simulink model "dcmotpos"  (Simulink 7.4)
settings: Solver=ode15s  StartTime=0.0  StopTime=0.1  MaxStep=1e-3  RelTol=1e-3

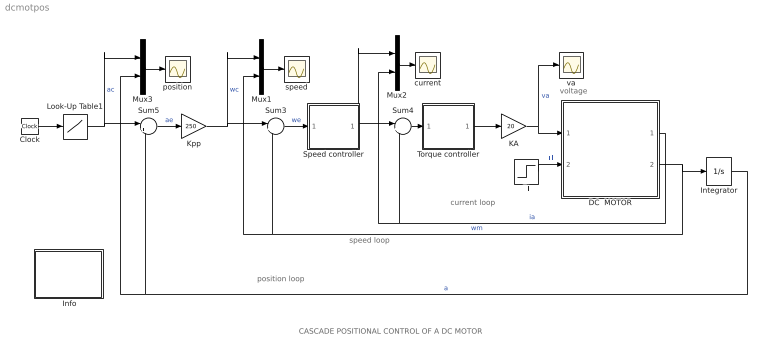
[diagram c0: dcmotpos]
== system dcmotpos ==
  note: voltage
  note: speed loop
  note: current loop
  note: position loop
  note: CASCADE POSITIONAL CONTROL OF A DC MOTOR
  " Info" : Subsystem
  Clock : Clock
  DC  MOTOR : Subsystem  mask{Ra=2.0, La=5.2e-3, J=1.5e-4, Bm=1e-3, K=0.1}
      mask prompts: Ra "Armature resistance [ohm]"; La "Armature inductance [H]"; J "Moment of inertia [Kg.m^2]"; Bm "Frictional torque cefficient"; K "Electromechanical coupling coefficient [N.m/A]"
      mask help: Block diagram of a dc motor with constant fiield excitation.
  Integrator : Integrator
  KA : Gain  Gain=20  ParameterDataType=sfix(16)  ParameterScaling=2^0  OutDataType=sfix(16)  OutScaling=2^0
  Kpp : Gain  Gain=250  ParameterDataType=sfix(16)  ParameterScaling=2^0  OutDataType=sfix(16)  OutScaling=2^0
  Look-Up Table1 : Lookup  InputValues="[0  .05  .05 1]"  Table="[1 1 .5  .5]"  OutDataType=sfix(16)  OutScaling=2^0
  Mux1 : Mux  Inputs=2
  Mux2 : Mux  Inputs=2
  Mux3 : Mux  Inputs=2
  Speed controller : Subsystem  mask{Kp=1.17, Ki=527, sat=18}
      mask prompts: Kp "Proportional gain (Kp)"; Ki "Integral gain (Ki)"; sat "Saturation limit [pu]"
      mask help: Proportional-Integral Speed Controller
  Sum3 : Sum  Inputs=|+-  OutDataType=sfix(16)  OutScaling=2^0
  Sum4 : Sum  Inputs=|+-  OutDataType=sfix(16)  OutScaling=2^0
  Sum5 : Sum  Inputs=|+-  OutDataType=sfix(16)  OutScaling=2^0
  Tl : Step  Time=0.04  After=0.38  SampleTime=0
  Torque controller : Subsystem  mask{Kp=1.38, Ki=5880, sat=3}
      mask prompts: Kp "Proportional gain (Kp)"; Ki "Integral gain (Ki)"; sat "Saturation limit [pu]"
      mask help: Proportional-Integral Speed Controller
  current : Scope
  position : Scope
  speed : Scope
  va : Scope
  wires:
  Tl/1 -> DC  MOTOR/2(Tl)  "Tl"
  Mux1/1 -> speed/1
  Mux2/1 -> current/1
  Kpp/1 -> Sum3/1, Mux1/1  "wc"
  DC  MOTOR/1(ia) -> Sum4/2, Mux2/2  "ia"
  Sum5/1 -> Kpp/1  "ae"
  Clock/1 -> Look-Up Table1/1
  Mux3/1 -> position/1
  Look-Up Table1/1 -> Sum5/1, Mux3/1  "ac"
  Integrator/1 -> Sum5/2, Mux3/2  "a"
  Speed controller/1(c) -> Sum4/1, Mux2/1
  Sum3/1 -> Speed controller/1(er)  "we"
  Sum4/1 -> Torque controller/1(er)
  Torque controller/1(c) -> KA/1
  KA/1 -> va/1, DC  MOTOR/1(va)  "va"
  DC  MOTOR/2(wm) -> Integrator/1, Sum3/2, Mux1/2  "wm"

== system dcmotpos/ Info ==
  note: This demo simulates the cascade control of a DC motor drive for position control

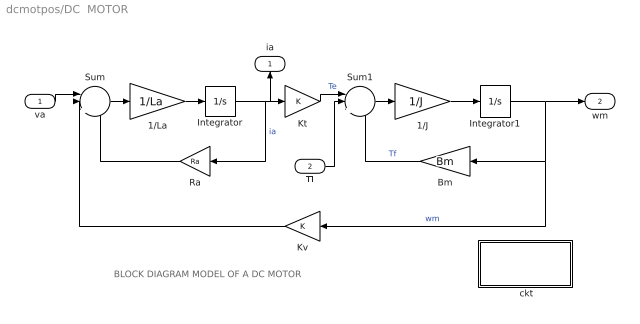
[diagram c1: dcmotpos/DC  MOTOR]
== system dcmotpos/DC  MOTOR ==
  note: BLOCK DIAGRAM MODEL OF A DC MOTOR
  va : Inport  OutDataType=sfix(16)  OutScaling=2^0
  Tl : Inport  Port=2  OutDataType=sfix(16)  OutScaling=2^0
  " ckt" : Subsystem
  1/J : Gain  Gain=1/J  ParameterDataType=sfix(16)  ParameterScaling=2^0  OutDataType=sfix(16)  OutScaling=2^0
  1/La : Gain  Gain=1/La  ParameterDataType=sfix(16)  ParameterScaling=2^0  OutDataType=sfix(16)  OutScaling=2^0
  Bm : Gain  Gain=Bm  ParameterDataType=sfix(16)  ParameterScaling=2^0  OutDataType=sfix(16)  OutScaling=2^0
  Integrator : Integrator
  Integrator1 : Integrator
  Kt : Gain  Gain=K  ParameterDataType=sfix(16)  ParameterScaling=2^0  OutDataType=sfix(16)  OutScaling=2^0
  Kv : Gain  Gain=K  ParameterDataType=sfix(16)  ParameterScaling=2^0  OutDataType=sfix(16)  OutScaling=2^0
  Ra : Gain  Gain=Ra  ParameterDataType=sfix(16)  ParameterScaling=2^0  OutDataType=sfix(16)  OutScaling=2^0
  Sum : Sum  Inputs=||+--  OutDataType=sfix(16)  OutScaling=2^0
  Sum1 : Sum  Inputs=||+--  OutDataType=sfix(16)  OutScaling=2^0
  ia : Outport
  wm : Outport  Port=2
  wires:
  Kv/1 -> Sum/2
  Ra/1 -> Sum/3
  Kt/1 -> Sum1/1  "Te"
  Bm/1 -> Sum1/3  "Tf"
  Sum/1 -> 1/La/1
  1/La/1 -> Integrator/1
  Integrator/1 -> Ra/1, Kt/1, ia/1  "ia"
  Sum1/1 -> 1/J/1
  1/J/1 -> Integrator1/1
  va/1 -> Sum/1
  Tl/1 -> Sum1/2
  Integrator1/1 -> Bm/1, Kv/1, wm/1  "wm"

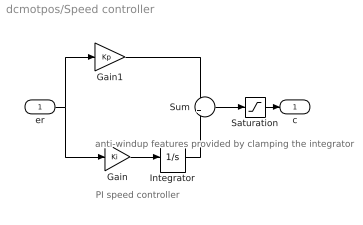
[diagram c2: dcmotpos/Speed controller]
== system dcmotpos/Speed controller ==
  note: anti-windup features provided by clamping the integrator
  note: PI speed controller
  er : Inport  OutDataType=sfix(16)  OutScaling=2^0
  Gain : Gain  Gain=Ki  ParameterDataType=sfix(16)  ParameterScaling=2^0  OutDataType=sfix(16)  OutScaling=2^0
  Gain1 : Gain  Gain=Kp  ParameterDataType=sfix(16)  ParameterScaling=2^0  OutDataType=sfix(16)  OutScaling=2^0
  Integrator : Integrator  LimitOutput=on  UpperSaturationLimit=sat  LowerSaturationLimit=-sat
  Saturation : Saturate  UpperLimit=sat  LowerLimit=-sat
  Sum : Sum  OutDataType=sfix(16)  OutScaling=2^0
  c : Outport  InitialOutput=0
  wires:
  Saturation/1 -> c/1
  Sum/1 -> Saturation/1
  er/1 -> Gain1/1, Gain/1
  Gain1/1 -> Sum/1
  Gain/1 -> Integrator/1
  Integrator/1 -> Sum/2

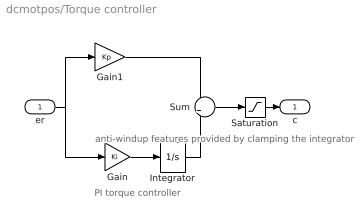
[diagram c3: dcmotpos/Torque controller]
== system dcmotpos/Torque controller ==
  note: anti-windup features provided by clamping the integrator
  note: PI torque controller
  er : Inport  OutDataType=sfix(16)  OutScaling=2^0
  Gain : Gain  Gain=Ki  ParameterDataType=sfix(16)  ParameterScaling=2^0  OutDataType=sfix(16)  OutScaling=2^0
  Gain1 : Gain  Gain=Kp  ParameterDataType=sfix(16)  ParameterScaling=2^0  OutDataType=sfix(16)  OutScaling=2^0
  Integrator : Integrator  LimitOutput=on  UpperSaturationLimit=sat  LowerSaturationLimit=-sat
  Saturation : Saturate  UpperLimit=sat  LowerLimit=-sat
  Sum : Sum  OutDataType=sfix(16)  OutScaling=2^0
  c : Outport  InitialOutput=0
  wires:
  Integrator/1 -> Sum/2
  Gain/1 -> Integrator/1
  Gain1/1 -> Sum/1
  er/1 -> Gain/1, Gain1/1
  Saturation/1 -> c/1
  Sum/1 -> Saturation/1

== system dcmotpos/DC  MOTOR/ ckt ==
